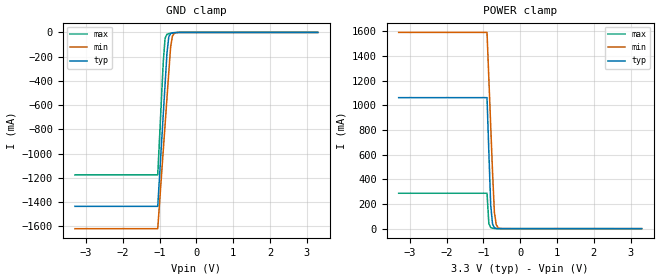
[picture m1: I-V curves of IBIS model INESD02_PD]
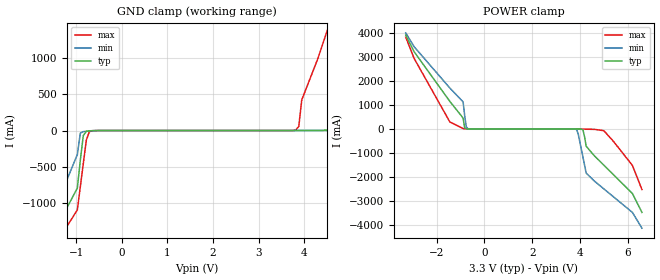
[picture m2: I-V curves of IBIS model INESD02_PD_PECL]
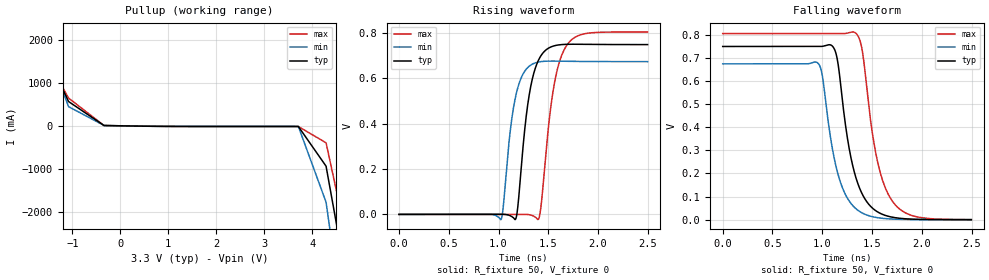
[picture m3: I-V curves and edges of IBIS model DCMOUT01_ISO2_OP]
|   This file is an IBIS representation of the   |
|   Integrated Device Technology, Inc.   |
|   ICS841604I   |
|   FEMTOCLOCKS CRYSTAL-TO-HCSL CLOCK GENERATOR   |
[IBIS Ver]   4.1
[File name]   841604i_3v3.ibs
[File Rev]   1.0
[Date]   2 Feb 2010
[Source]   Originated at Integrated Device Technology, Inc.
[Disclaimer]
IDT hereby grants the user of this IBIS model a non-exclusive,
nontransferable license to use this IBIS model under the following terms.
Before using this IBIS model, the user should read this license.
If the user does not accept these terms,  the IBIS model should be
returned to IDT within 30 days.
   The user is granted this license only to use the IBIS model and
is not granted rights to sell, load, rent, lease or license the IBIS
model in whole or in part, or in modified form to anyone other than
user. User may modify the IBIS model to suit its specific
applications but rights to derivative works and such modifications
shall belong to IDT.
   This IBIS model is provided on an "AS IS" basis and IDT makes
absolutely no warranty with respect to the information contained
herein. IDT DISCLAIMS AND CUSTOMER WAIVES ALL WARRANTIES, EXPRESS
OR IMPLIED, INCLUDING WARRANTIES OF MERCHANTABILITY OR FITNESS FOR
A PARTICULAR PURPOSE. The entire risk as to quality and performance
is with the Customer. ACCORDINGLY, IN NO EVENT SHALL THE COMPANY BE
LIABLE FOR ANY DAMAGES, WHETHER IN CONTRACT OR TORT,INCLUDING ANY
LOST PROFITS OR OTHER INCIDENTAL, CONSEQUENTIAL, EXEMPLARY, OR
PUNITIVE DAMAGES ARISING OUT OF THE USE OR APPLICATION OF THE IBIS
model provided in this package. Further, IDT reserves the right to
make changes without notice to any product herein to improve
reliability, function, or design. IDT does not convey any license
under patent rights or any other intellectual property rights,
including those of third parties.
   IDT is not obligated to provide maintenance or support
for the licensed IBIS model.
[Copyright]   Copyright 2008 by Integrated Device Technology, Inc.
[Component]   841604AGI
[Manufacturer] Integrated Device Technology, Inc.
[Package]
|TSSOP 28 Lead
|   typ   min   max
R_pkg   60.65m   52.4m   68.9m
L_pkg   1.989nH   1.431nH   2.547nH
C_pkg   0.314pF   0.254pF   0.374pF
[Pin]   signal_name   model_name   R_pin   L_pin   C_pin
1   REF_SEL   INESD02_PD   68.9m   2.547n   0.374p
2   REF_IN   INESD02_PD_PECL   66.2m   2.360n   0.254p
3   VDD   POWER   63.4m   2.174n   0.334p
4   GND   GND   60.6m   1.988n   0.314p
5   XTAL_IN   NC   57.9m   1.802n   0.294p
6   XTAL_OUT   NC   55.1m   1.616n   0.274p
7   MR_nOE   INESD02_PD   52.4m   1.431n   0.254p
8   VDD   POWER   52.4m   1.431n   0.254p
9   NC   NC   55.1m   1.616n   0.274p
10   NC   NC   57.9m   1.802n   0.294p
11   NC   NC   60.6m   1.988n   0.314p
12   NC   NC   63.4m   2.174n   0.334p
13   GND   GND   66.2m   2.360n   0.254p
14   VDD   POWER   68.9m   2.547n   0.374p
15   Q0   DCMOUT01_ISO2_OP   68.9m   2.547n   0.374p
16   nQ0   DCMOUT01_ISO2_OP   66.2m   2.360n   0.254p
17   Q1   DCMOUT01_ISO2_OP   63.4m   2.174n   0.334p
18   nQ1   DCMOUT01_ISO2_OP   60.6m   1.988n   0.314p
19   GND   GND   57.9m   1.802n   0.294p
20   Q2   DCMOUT01_ISO2_OP   55.1m   1.616n   0.274p
21   nQ2   DCMOUT01_ISO2_OP   52.4m   1.431n   0.254p
22   Q3   DCMOUT01_ISO2_OP   52.4m   1.431n   0.254p
23   nQ3   DCMOUT01_ISO2_OP   55.1m   1.616n   0.274p
24   VDD   POWER   57.9m   1.802n   0.294p
25   FSEL   INESD02_PD   60.6m   1.988n   0.314p
26   IREF   NC   63.4m   2.174n   0.334p
27   BYPASS   INESD02_PD   66.2m   2.360n   0.254p
28   VDDA   POWER   68.9m   2.547n   0.374p
[Diff Pin]  inv_pin  vdiff tdelay_typ tdelay_min  tdelay_max
15   16   NA   0   0   0
17   18   NA   0   0   0
20   21   NA   0   0   0
22   23   NA   0   0   0
| Models and submodels in the file (3): INESD02_PD (Input), INESD02_PD_PECL (Input), DCMOUT01_ISO2_OP (Open_source)
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[Model]   INESD02_PD
Model_type   Input
Polarity   Non-Inverting
Vinl = 0.80V
Vinh = 2.0V
|   typ   min   max
C_comp   2pF   1.5pF   2.5pF
|   typ   min   max
[Voltage range]  3.3V   3.15V   3.45V
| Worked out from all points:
|   GND clamp passes 1 mA (typ) near -0.56 V on its own axis
|   POWER clamp passes 1 mA (typ) near -0.61 V on its own axis
[GND_clamp]
|Voltage   I(typ)   I(min)   I(max)
-3.3V     -1.436A    -1.62A     -1.176A
-1.05V    -1.436A    -1.62A     -1.176A
-900mV    -678.5mA   -975.1mA   -244mA
-850mV    -426.1mA   -760.1mA   -46.85mA
-800mV    -173.9mA   -545.4mA   -16.11mA
-750mV    -36.96mA   -330.7mA   -9.916mA
-700mV    -9.696mA   -120.2mA   -7.056mA
-650mV    -3.545mA   -29.7mA    -4.857mA
-600mV    -1.629mA   -7.52mA    -3.049mA
-400mV    -52.81uA   -52.52uA   -108.7uA
3.3V      71.13uA    77.43uA    62.11uA
[POWER_clamp]
|Voltage   I(typ)   I(min)   I(max)
-3.3V     1.063A     1.593A     287.3mA
-900mV    1.063A     1.593A     287.3mA
-850mV    620.5mA    1.215A     41.84mA
-800mV    191.6mA    837.5mA    8.757mA
-750mV    37.76mA    460.2mA    3.328mA
-700mV    8.104mA    133.8mA    1.728mA
-650mV    2.076mA    32.66mA    905.3uA
-600mV    678.1uA    8.083mA    443.8uA
-450mV    104.2uA    213.3uA    89.09uA
3.3V      -3.041nA   -3.986uA   0A
[Model]   INESD02_PD_PECL
Model_type  Input
Polarity   Non-Inverting
Vinl = 0.8V
Vinh = 2.0V
|   typ   min   max
C_comp   2pF   1.5pF   2.5pF
|   typ   min   max
[Voltage range]  3.3V   3.15V   3.45V
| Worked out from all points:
|   GND clamp passes 1 mA (typ) near -0.59 V on its own axis
|   POWER clamp passes 1 mA (typ) near -0.70 V on its own axis
[GND_clamp]
-3.3V     -3.894A    -4.294A    -3.674A
-1.6V     -1.569A    -1.322A    -1.74A
-974.8mV  -794.1mA   -331.5mA   -1.096A
-843.4mV  -68.33mA   -15.34mA   -452.9mA
-646.5mV  -1.912mA   -4.151mA   -2.665mA
3.818V    89.38uA    70.49uA    7.198mA
3.95V     342.2uA    75.94uA    423.8mA
4.6V      7.437mA    165.5uA    1.553A
4.9V      78.32mA    440.9uA    2.118A
5.5V      1.293A     2.769mA    3.249A
6.25V     2.651A     112.4mA    4.38A
6.6V      3.331A     896.1mA    4.946A
[POWER_clamp]
-3.3V     3.923A     4.017A     3.838A
-2.95V    3.23A      3.44A      2.951A
-1.45V    1.149A     1.709A     289.6mA
-896.9mV  456.5mA    1.133A     15.4mA
-762.9mV  4.223mA    91.07mA    1.486mA
-695.9mV  792.2uA    10.73mA    555.6uA
3.861V    -556.7uA   -26.14mA   -39.45uA
4.129V    -41.85mA   -1.19A     -4.904mA
4.263V    -724.2mA   -1.847A    -12.04mA
5V        -1.514A    -2.505A    -71.38mA
6.2V      -2.701A    -3.492A    -1.525A
6.6V      -3.492A    -4.151A    -2.536A
[Model]   DCMOUT01_ISO2_OP
Model_type   Open_source
Polarity   Non-Inverting
|   typ   min   max
C_comp   2pF   1.5pF   2.5pF
Vmeas = .344V
Rref = 50
Cref = 0
Vref = 0V
|   typ   min   max
[Voltage range]   3.3V   3.135V   3.465V
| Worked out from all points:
|   slope of the pullup table from 0 to 0.495 V, typ, clamps not added: 54.5 ohm
|   rising waveform, R_fixture 50, V_fixture 0: 20-80 % time 123ps typ, 114ps min, 139ps max; typ from 0 V to 0.749 V
|   falling waveform, R_fixture 50, V_fixture 0: 20-80 % time 182ps typ, 179ps min, 184ps max; typ from 0.749 V to 0 V
[Pullup]
|Voltage   I (typ)   I (min)   I (max)
-3.3V     5.929A     7.281A     5.128A
-2.56V    4.138A     5A         3.631A
-1.82V    2.349A     2.722A     2.136A
-1.08V    565.7mA    446.7mA    647.1mA
-340mV    7.268mA    8.174mA    6.641mA
3.71V     -15.08mA   -14.13mA   -16.17mA
4.288V    -939.9mA   -1.778A    -395.8mA
4.866V    -4.531A    -6.361A    -3.386A
6.6V      -15.32A    -20.11A    -12.39A
[Ramp]
|   typ   min   max
dV/dt_r   0.618/0.195n   0.559/0.181n   0.661/0.221n
dV/dt_f   0.605/0.294n   0.545/0.287n   0.649/0.3n
R_load =   50.0000
[Rising Waveform]
R_fixture = 50
V_fixture = 0
V_fixture_max = 0
V_fixture_min = 0
C_fixture = 0.0p
| Time   typ   min   max
0s        1.469nV    329.3pV    95.28nV
1.026ns   401.4uV    -22.55mV   617.5nV
1.119ns   -5.95mV    370.6mV    -10.36uV
1.171ns   -21.47mV   518.2mV    2.251uV
1.294ns   484.8mV    647.9mV    -448.4uV
1.399ns   677.8mV    671.8mV    -22.17mV
1.429ns   701.6mV    674mV      42.96mV
1.547ns   741.9mV    676.3mV    539.5mV
1.672ns   750mV      675.5mV    736mV
2.498ns   748.9mV    673.8mV    804.6mV
[Falling Waveform]
R_fixture = 50
V_fixture = 0
V_fixture_max = 0
V_fixture_min = 0
C_fixture = 0.0p
| Time   typ   min   max
0s        748.9mV    673.8mV    804.6mV
953.5ps   748.5mV    678.1mV    804.6mV
1.001ns   749.6mV    621.8mV    804.6mV
1.101ns   750.8mV    308.7mV    804.7mV
1.154ns   687.2mV    203.9mV    804.5mV
1.334ns   187.9mV    49.06mV    807.6mV
1.401ns   111mV      28.85mV    732.3mV
1.549ns   35.42mV    9.066mV    263.9mV
1.689ns   12.05mV    3.027mV    89.91mV
2.498ns   24.47uV    5.43uV     200.3uV
